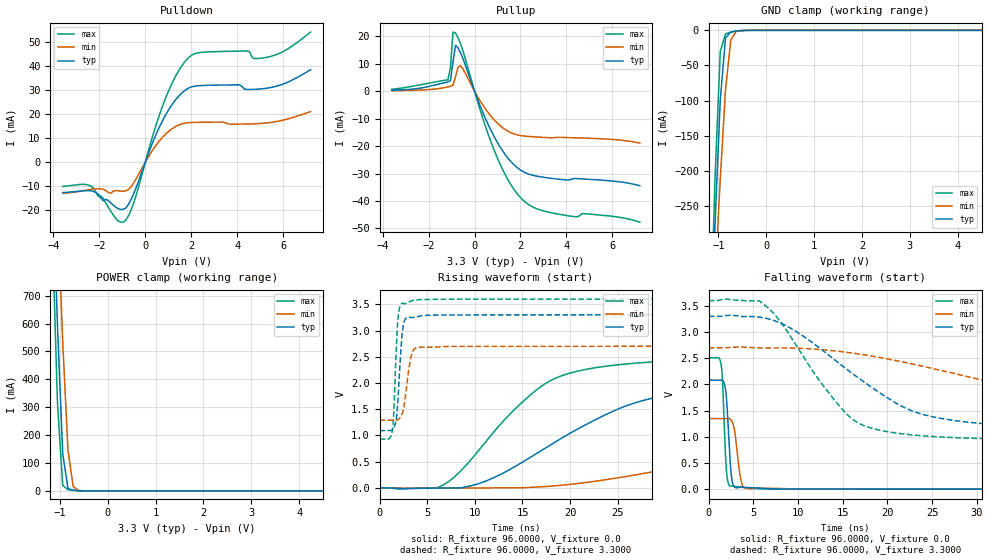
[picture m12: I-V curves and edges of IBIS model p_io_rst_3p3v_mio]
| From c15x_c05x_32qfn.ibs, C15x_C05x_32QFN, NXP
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[Model] p_io_rst_3p3v_mio
|   Model p_io_rst_3p3v_mio
| This model was characterised for following simulation conditions:
| External (pad) voltage:
|   - Typ: 3.3V,   - Min: 2.7V,   - Max: 3.6V
| Library cells for typ/min/max conditions are connected as defined below:
|  pad - External Pad
|  ipp_do_lv - Core Input
|  ipp_obe_lv - Output Buffer Enable
|  IOGC - NC
|  REFH3V3 - REFH3V3
|  REFL3V3 - REFL3V3
|  ZI - NC
|  abut_ncal_vddio[1] - vddio
|  abut_ncal_vddio[2] - vddio
|  abut_ncal_vddio[3] - vssio
|  abut_ncal_vddio[4] - vddio
|  abut_ncal_vddio[5] - vddio
|  abut_ncal_vddio[6] - vssio
|  abut_pcal_vddio[1] - vssio
|  abut_pcal_vddio[2] - vssio
|  abut_pcal_vddio[3] - vddio
|  abut_pcal_vddio[4] - vssio
|  abut_pcal_vddio[5] - vssio
|  abut_pcal_vddio[6] - vddio
|  ipp_do_1p8v - ipp_do_1p8v
|  ipp_eftd_lv - NC
|  ipp_ina_mux_vddio - NC
|  ipp_ina_mux_vddio[0] - NC
|  ipp_ina_mux_vddio[1] - NC
|  ipp_ina_r0_vddio - NC
|  ipp_ina_r0a_vddio - NC
|  ipp_ina_r0b_vddio - NC
|  ipp_ina_r0c_vddio - NC
|  ipp_ina_r0d_vddio - NC
|  ipp_ina_r0e_vddio - NC
|  ipp_ina_r0f_vddio - NC
|  ipp_ina_r300_vddio - NC
|  ipp_ina_r300a_vddio - NC
|  ipp_ina_r300b_vddio - NC
|  ipp_ina_r300c_vddio - NC
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Model_type I/O
Polarity   Non-Inverting
Enable   Active-High
Vinl =   0.9900V
Vinh =   2.3100V
Vmeas =  1.6500V
Cref =   30.0000pF
Rref =   1.0000M
Vref =   3.3000V
C_comp   1.3413pF   1.2954pF   1.4090pF
|C_comp_pullup   0.5415pF   0.5708pF   0.5218pF
|C_comp_pulldown   0.7061pF   0.7464pF   0.6762pF
[Model Spec]
| variable   typ   min   max
Vinh   2.3100V   1.8900V   2.5200V
Vinl   0.9900V   0.8100V   1.0800V
[Temperature Range]   25.0000   0.1250k   -40.0000
[Voltage Range]   3.3000V   2.7000V   3.6000V
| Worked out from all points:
|   slope of the pulldown table from 0 to 0.495 V, typ, clamps not added: 40.8 ohm
|   slope of the pullup table from 0 to 0.495 V, typ, clamps not added: 47.8 ohm
|   GND clamp passes 1 mA (typ) near -0.63 V on its own axis
|   POWER clamp passes 1 mA (typ) near -0.62 V on its own axis
|   rising waveform, R_fixture 96.0000, V_fixture 0.0: 20-80 % time 13.3ns typ, 27.9ns min, 8.15ns max; typ from 0 V to 2.08 V
|   rising waveform, R_fixture 96.0000, V_fixture 3.3000: 20-80 % time 452ps typ, 631ps min, 368ps max; typ from 1.09 V to 3.3 V
|   falling waveform, R_fixture 96.0000, V_fixture 0.0: 20-80 % time 424ps typ, 578ps min, 358ps max; typ from 2.08 V to 0 V
|   falling waveform, R_fixture 96.0000, V_fixture 3.3000: 20-80 % time 11.1ns typ, 24.1ns min, 6.71ns max; typ from 3.3 V to 1.09 V
[Pulldown]
|Voltage   I(typ)   I(min)   I(max)
-3.6V     -12.69mA   -13mA      -10.11mA
-2.39V    -11.94mA   -11.39mA   -9.907mA
-1.29V    -18.76mA   -11.81mA   -23.45mA
-960mV    -19.66mA   -12.1mA    -25.04mA
-520mV    -13.49mA   -8.854mA   -17.41mA
800mV     18.21mA    10.89mA    24.66mA
1.35V     26.41mA    15.03mA    36.46mA
1.79V     30.37mA    16.39mA    42.68mA
3V        32.13mA    16.71mA    46.1mA
4.43V     30.33mA    15.91mA    46.4mA
5.31V     30.89mA    16.4mA     43.78mA
7.2V      38.58mA    21.1mA     54.28mA
[Pullup]
|Voltage   I(typ)   I(min)   I(max)
-3.6V     377.2uA    207.6uA    732.6uA
-1.16V    3.394mA    1.601mA    4.181mA
-1.05V    3.923mA    1.815mA    8.669mA
-940mV    10.63mA    2.206mA    21.56mA
-830mV    16.69mA    5.218mA    21.23mA
-720mV    15.82mA    8.857mA    19.48mA
-610mV    14mA       9.299mA    17.3mA
820mV     -16.02mA   -10.13mA   -20.76mA
1.48V     -24.66mA   -14.68mA   -32.62mA
2.03V     -28.88mA   -16.19mA   -39.03mA
3.46V     -31.87mA   -16.93mA   -44.5mA
7.2V      -34.47mA   -18.93mA   -47.74mA
[GND_clamp]
|Voltage   I(typ)   I(min)   I(max)
-3.6V     -5.607A    -4.475A    -7.131A
-1.18V    -473.1mA   -501.9mA   -466.9mA
-1.07V    -276.4mA   -353.7mA   -210.9mA
-960mV    -99.46mA   -211.8mA   -30.01mA
-850mV    -10.76mA   -84.44mA   -5.071mA
-740mV    -2.289mA   -13.69mA   -2.754mA
-630mV    -1.015mA   -1.69mA    -1.169mA
-520mV    -313.8uA   -442.2uA   -284uA
7.2V      0A         0A         0A
[POWER_clamp]
|Voltage   I(typ)   I(min)   I(max)
-3.6V     14.37A     12.86A     16.2A
-1.16V    1.168A     1.525A     943.2mA
-1.05V    594.1mA    1.025A     315.9mA
-940mV    133.7mA    534mA      20.04mA
-830mV    8.718mA    144.9mA    4.268mA
-720mV    2.135mA    15.37mA    2.235mA
-610mV    851.7uA    1.853mA    843.3uA
7.2V      0A         0A         0A
[Ramp]
| variable   typ   min   max
dV/dt_r  1.2491/13.3334n   0.8005/27.8739n   1.5061/8.1549n
dV/dt_f  1.3249/11.0982n   0.8410/24.1325n   1.6025/6.7094n
R_load = 96.0000
[Rising Waveform]
R_fixture= 96.0000
V_fixture= 0.0
V_fixture_min= 0.0
V_fixture_max= 0.0
|time   V(typ)   V(min)   V(max)
0s        3.039nV    105.4nV    10.42nV
6.64ns    -4.375mV   -3.103mV   51.98mV
11.15ns   129.6mV    -1.763mV   880.6mV
17.18ns   735.2mV    22.52mV    1.962V
20.38ns   1.081V     74.48mV    2.208V
25.51ns   1.538V     206.2mV    2.356V
36.74ns   1.902V     580.1mV    2.462V
48.64ns   2.005V     942.9mV    2.494V
60.18ns   2.046V     1.127V     2.504V
132.1ns   2.082V     1.334V     2.51V
[Rising Waveform]
R_fixture= 96.0000
V_fixture= 3.3000
V_fixture_min= 2.7000
V_fixture_max= 3.6000
|time   V(typ)   V(min)   V(max)
0s        1.092V     1.289V     929.2mV
1.36ns    1.111V     1.289V     1.105V
1.486ns   1.142V     1.288V     1.398V
1.793ns   1.349V     1.29V      2.801V
2.12ns    2.276V     1.332V     3.447V
2.363ns   2.915V     1.408V     3.517V
2.594ns   3.172V     1.585V     3.513V
3.276ns   3.249V     2.476V     3.56V
3.908ns   3.264V     2.674V     3.585V
132.1ns   3.3V       2.7V       3.6V
[Falling Waveform]
R_fixture= 96.0000
V_fixture= 0.0
V_fixture_min= 0.0
V_fixture_max= 0.0
|time   V(typ)   V(min)   V(max)
0s        2.082V     1.348V     2.51V
1.39ns    2.083V     1.348V     2.371V
1.553ns   2.074V     1.348V     2.033V
1.829ns   1.951V     1.348V     808.8mV
1.976ns   1.756V     1.348V     356.2mV
2.422ns   455.2mV    1.334V     58.45mV
2.765ns   70.11mV    1.215V     54.89mV
3.656ns   36.15mV    136.4mV    40.55mV
4.378ns   32.26mV    10.24mV    26.67mV
132.1ns   454.1nV    7.099uV    34.9nV
[Falling Waveform]
R_fixture= 96.0000
V_fixture= 3.3000
V_fixture_min= 2.7000
V_fixture_max= 3.6000
|time   V(typ)   V(min)   V(max)
0s        3.3V       2.7V       3.6V
5.746ns   3.284V     2.698V     3.585V
9.611ns   3.03V      2.694V     2.796V
15.72ns   2.254V     2.608V     1.389V
17.99ns   1.974V     2.55V      1.176V
21.86ns   1.562V     2.425V     1.053V
31.29ns   1.243V     2.056V     963.4mV
41.64ns   1.156V     1.678V     940.2mV
52.45ns   1.122V     1.493V     933.2mV
132.1ns   1.092V     1.298V     929.2mV
